PROGRAM MAIN

VAR
	bEnable: BOOL := TRUE;				(*enable or disable the functionblock by changing the value of this variable*)
	fbOcaDevice: FB_OcaDevice;			(*instance of the function block which represents the OCA Device*)
	fbOcaGain: ARRAY[E_Channel.A ..E_Channel.D] OF FB_OcaGain;	(*instances of the function block which represents the OCA Object*)

	{attribute hide}	bInit: BOOL;	(*will be TRUE after the first cycle*) 

	stRole: ARRAY[E_Channel.A ..E_Channel.D] OF ST_StringProperty;			(*structures which will contain the result 'Role' *)
	stLabel: ARRAY[E_Channel.A ..E_Channel.D] OF ST_StringProperty;			(*structures which will contain the text of the property 'Label' *)
	stGain:  ARRAY[E_Channel.A ..E_Channel.D] OF ST_Float32Property;		(*structures which will contain the value of the property 'Gain'*)
	aNewValueGain: ARRAY[E_Channel.A ..E_Channel.D] OF REAL;				(*the values which sould be set*)
	_aNewValueGain: ARRAY[E_Channel.A ..E_Channel.D] OF REAL;

	eCurrentChannel: E_Channel;		(*variable used to loop throug all channels*) 	
END_VAR

A_Init();		(*enter IP Address and other parameters of the device in this Action*)  
A_Operation();	(*calls FB_OcaDevice and the Subscription Method*) 
A_Operation1();	(*tries to get basic, inherited properties and call the method GetGain*)
A_Operation2();	(*tries to read Notifications*)
A_Operation3();	(*tries to set new 'Gain'-values*)

ACTION A_Init:
IF NOT bInit THEN
	bInit := TRUE;

	(* ----------- Init devices -------------*)
	InitDeviceList();
	fbOcaDevice.sDeviceName := 'Amplifier_2';

	fbOcaDevice.bLocalOcaDevice := FALSE;

	
	(* ----------- Init the object (assigned to a device) -------------*)
	InitOcaObjectList();
	fbOcaGain[E_Channel.A].__setsOcaObjectDescription(sOcaObjectDescription := 'Gain_A', pLink := fbOcaDevice.pLink); 
	fbOcaGain[E_Channel.B].__setsOcaObjectDescription(sOcaObjectDescription := 'Gain_B', pLink := fbOcaDevice.pLink); 
	fbOcaGain[E_Channel.C].__setsOcaObjectDescription(sOcaObjectDescription := 'Gain_C', pLink := fbOcaDevice.pLink); 
	fbOcaGain[E_Channel.D].__setsOcaObjectDescription(sOcaObjectDescription := 'Gain_D', pLink := fbOcaDevice.pLink); 
END_IF
END_ACTION

ACTION A_Operation:
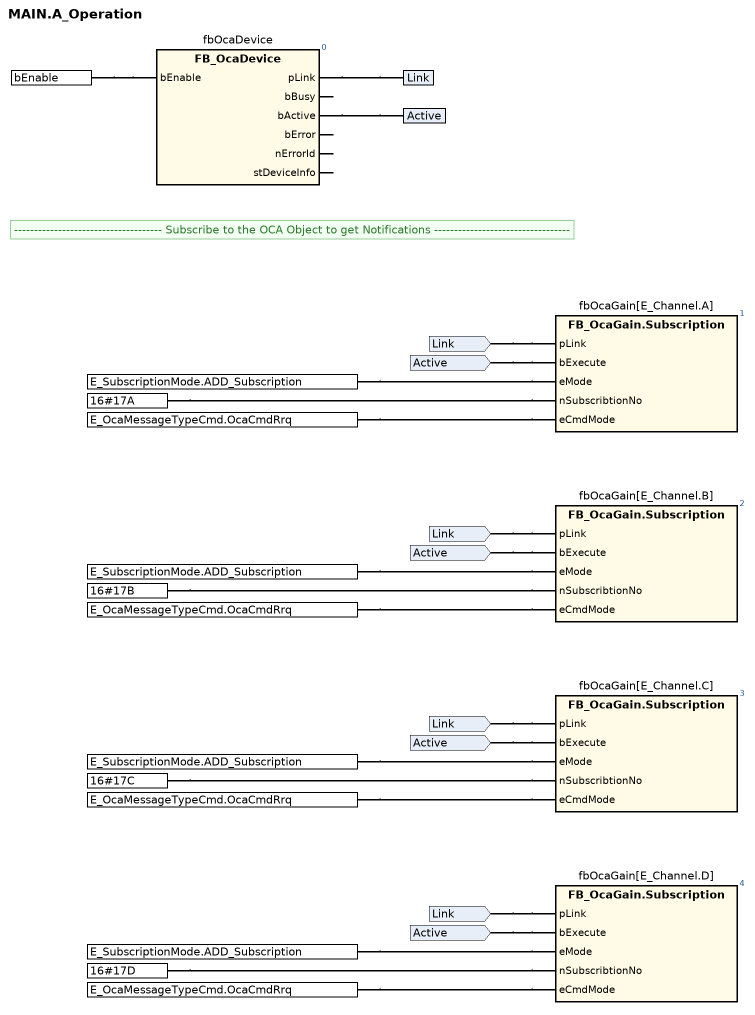
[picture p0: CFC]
fbOcaDevice(bEnable := bEnable); // FB_OcaDevice
// ------------------------------------- Subscribe to the OCA Object to get Notifications ----------------------------------
fbOcaGain[E_Channel.A].Subscription(pLink := fbOcaDevice.pLink, bExecute := fbOcaDevice.bActive, eMode := E_SubscriptionMode.ADD_Subscription, nSubscribtionNo := 16#17A, eCmdMode := E_OcaMessageTypeCmd.OcaCmdRrq);
fbOcaGain[E_Channel.B].Subscription(pLink := fbOcaDevice.pLink, bExecute := fbOcaDevice.bActive, eMode := E_SubscriptionMode.ADD_Subscription, nSubscribtionNo := 16#17B, eCmdMode := E_OcaMessageTypeCmd.OcaCmdRrq);
fbOcaGain[E_Channel.C].Subscription(pLink := fbOcaDevice.pLink, bExecute := fbOcaDevice.bActive, eMode := E_SubscriptionMode.ADD_Subscription, nSubscribtionNo := 16#17C, eCmdMode := E_OcaMessageTypeCmd.OcaCmdRrq);
fbOcaGain[E_Channel.D].Subscription(pLink := fbOcaDevice.pLink, bExecute := fbOcaDevice.bActive, eMode := E_SubscriptionMode.ADD_Subscription, nSubscribtionNo := 16#17D, eCmdMode := E_OcaMessageTypeCmd.OcaCmdRrq);
END_ACTION

ACTION A_Operation1:
(*loop to all Channels (A,B,C,D) to get the Property 'Role', the Property 'Label'  and the current value of 'Gain' - this is done just once cause of the rising edge at bExecute*)
FOR eCurrentChannel := E_Channel.A TO E_Channel.D DO
	fbOcaGain[eCurrentChannel].GetRole(
		pLink:= fbOcaDevice.pLink,						//link the OCA Object to the OCA Device
		bExecute:= fbOcaDevice.bActive);				//execute this methode when the instance of FB_OcaDevice is ready and do this just once to get the current Role of the OCA Object
	stRole[eCurrentChannel] := fbOcaGain[eCurrentChannel].stRole;	

	fbOcaGain[eCurrentChannel].GetLabel(
		pLink:= fbOcaDevice.pLink,						//link the OCA Object to the OCA Device
		bExecute:= fbOcaDevice.bActive);				//execute this methode when the instance of FB_OcaDevice is ready and do this just once to get the current Label of the OCA Object
	stLabel[eCurrentChannel] := fbOcaGain[eCurrentChannel].stLabel;	

	fbOcaGain[eCurrentChannel].GetGain(
		pLink:= fbOcaDevice.pLink,						//link the OCA Object to the OCA Device
		bExecute:= fbOcaDevice.bActive);				//execute this methode when the instance of FB_OcaDevice is ready and do this just once to get the current Label of the OCA Object
	stGain[eCurrentChannel] := fbOcaGain[eCurrentChannel].stGain;	
END_FOR
END_ACTION

ACTION A_Operation2:
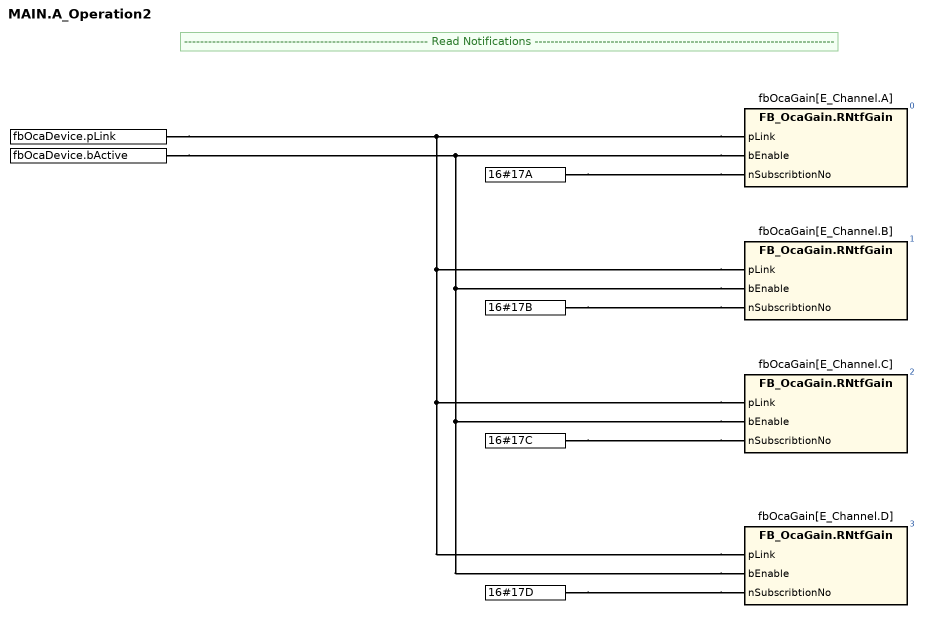
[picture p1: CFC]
// ------------------------------------------------------------- Read Notifications ---------------------------------------------------------------------------
fbOcaGain[E_Channel.A].RNtfGain(pLink := fbOcaDevice.pLink, bEnable := fbOcaDevice.bActive, nSubscribtionNo := 16#17A);
fbOcaGain[E_Channel.B].RNtfGain(pLink := fbOcaDevice.pLink, bEnable := fbOcaDevice.bActive, nSubscribtionNo := 16#17B);
fbOcaGain[E_Channel.C].RNtfGain(pLink := fbOcaDevice.pLink, bEnable := fbOcaDevice.bActive, nSubscribtionNo := 16#17C);
fbOcaGain[E_Channel.D].RNtfGain(pLink := fbOcaDevice.pLink, bEnable := fbOcaDevice.bActive, nSubscribtionNo := 16#17D);
END_ACTION

ACTION A_Operation3:
(*loop to all Channels (A,B,C,D) to possibly set new 'Gain' values*)
FOR eCurrentChannel := E_Channel.A TO E_Channel.D DO
	(*Set the Gain Property*)
	fbOcaGain[eCurrentChannel].SetGain(
		pLink:= fbOcaDevice.pLink,						//link the OCA Object to the OCA Device
		bExecute:= 
				(_aNewValueGain[eCurrentChannel] <> aNewValueGain[eCurrentChannel]) 
				AND fbOcaDevice.bActive,				//only execute this methode if the value changes
		fGain:= aNewValueGain[eCurrentChannel], 
		eCmdMode:= E_OcaMessageTypeCmd.OcaCmd);			//no response required - subscribed to get notifications! 					 
		
	
	_aNewValueGain[eCurrentChannel] := SEL(fbOcaDevice.bActive,
 											_aNewValueGain[eCurrentChannel],
											aNewValueGain[eCurrentChannel]);	 
	stGain[eCurrentChannel] := fbOcaGain[eCurrentChannel].stGain;	
END_FOR
END_ACTION

(* set parameters of the device *)
METHOD InitDeviceList
VAR
	i: INT  (0..(GVL_AES70.MAX_DEVICES - 1)) := 0;	//variable only used to count during initialization  
END_VAR

GVL_AES70.aOcaDevices[i].ipAddr := '169.254.40.175';		// the ip addres of the first device
GVL_AES70.aOcaDevices[i].ipPort := 30013;				// the port of the first device
GVL_AES70.aOcaDevices[i].sDeviceName := 'Amplifier_1';	// the unique name of the first device 

i:=i+1;
GVL_AES70.aOcaDevices[i].ipAddr := '169.254.1.7';	// the ip addres of the second device
GVL_AES70.aOcaDevices[i].ipPort := 30013;				// the port of the second device
GVL_AES70.aOcaDevices[i].sDeviceName := 'Amplifier_2';	// the unique name of the second device 

i:=i+1;
GVL_AES70.aOcaDevices[i].ipAddr := '169.254.163.144';	// the ip addres of the third device
GVL_AES70.aOcaDevices[i].ipPort := 42502;				// the port of the third device
GVL_AES70.aOcaDevices[i].sDeviceName := 'Amplifier_3';	// the unique name of the third device
END_METHOD

(* set parameters of the objects *)
METHOD InitOcaObjectList
VAR
	i: 	UINT  (0..(GVL_AES70.MAX_DEVICES - 1)) := 0;				//variable only used to count during initialization
	ii: UINT  (0..(GVL_AES70.MAX_OBJECTS_PER_DEVICE - 1)) := 0;		//variable only used to count during initialization  
END_VAR
(*Objects used by the first device*)
ii := 0;
GVL_AES70.aOcaDevices[i].aOcaObjectList[ii].nOcaObjectNr := 16#10000100;
GVL_AES70.aOcaDevices[i].aOcaObjectList[ii].nOwnerNr := 16#10001FE;
GVL_AES70.aOcaDevices[i].aOcaObjectList[ii].sDescription := 'PwrOn';
ii := ii+1;
GVL_AES70.aOcaDevices[i].aOcaObjectList[ii].nOcaObjectNr := 16#10000101;
GVL_AES70.aOcaDevices[i].aOcaObjectList[ii].nOwnerNr := 16#10001FE;
GVL_AES70.aOcaDevices[i].aOcaObjectList[ii].sDescription := 'LockCmd';
ii := ii+1;
GVL_AES70.aOcaDevices[i].aOcaObjectList[ii].nOcaObjectNr := 16#10000102;
GVL_AES70.aOcaDevices[i].aOcaObjectList[ii].nOwnerNr := 16#10001FE;
GVL_AES70.aOcaDevices[i].aOcaObjectList[ii].sDescription := 'Buzzer';
ii := ii+1;
GVL_AES70.aOcaDevices[i].aOcaObjectList[ii].nOcaObjectNr := 16#10000103;
GVL_AES70.aOcaDevices[i].aOcaObjectList[ii].nOwnerNr := 16#10001FE;
GVL_AES70.aOcaDevices[i].aOcaObjectList[ii].sDescription := 'LockScreen';
ii := ii+1;
GVL_AES70.aOcaDevices[i].aOcaObjectList[ii].nOcaObjectNr := 16#1000010F;
GVL_AES70.aOcaDevices[i].aOcaObjectList[ii].nOwnerNr := 16#10001FE;
GVL_AES70.aOcaDevices[i].aOcaObjectList[ii].sDescription := 'InputModes';
ii := ii+1;
GVL_AES70.aOcaDevices[i].aOcaObjectList[ii].nOcaObjectNr := 16#10000111;
GVL_AES70.aOcaDevices[i].aOcaObjectList[ii].nOwnerNr := 16#10001FE;
GVL_AES70.aOcaDevices[i].aOcaObjectList[ii].sDescription := 'OutputMode';
ii := ii+1;
GVL_AES70.aOcaDevices[i].aOcaObjectList[ii].nOcaObjectNr := 16#10008205;
GVL_AES70.aOcaDevices[i].aOcaObjectList[ii].nOwnerNr := 16#10002FE;
GVL_AES70.aOcaDevices[i].aOcaObjectList[ii].sDescription := 'Mute_A';
ii := ii+1;
GVL_AES70.aOcaDevices[i].aOcaObjectList[ii].nOcaObjectNr := 16#10010205;
GVL_AES70.aOcaDevices[i].aOcaObjectList[ii].nOwnerNr := 16#10002FE;
GVL_AES70.aOcaDevices[i].aOcaObjectList[ii].sDescription := 'Mute_B';
ii := ii+1;
GVL_AES70.aOcaDevices[i].aOcaObjectList[ii].nOcaObjectNr := 16#10018205;
GVL_AES70.aOcaDevices[i].aOcaObjectList[ii].nOwnerNr := 16#10002FE;
GVL_AES70.aOcaDevices[i].aOcaObjectList[ii].sDescription := 'Mute_C';
ii := ii+1;
GVL_AES70.aOcaDevices[i].aOcaObjectList[ii].nOcaObjectNr := 16#10020205;
GVL_AES70.aOcaDevices[i].aOcaObjectList[ii].nOwnerNr := 16#10002FE;
GVL_AES70.aOcaDevices[i].aOcaObjectList[ii].sDescription := 'Mute_D';
ii := ii+1;
GVL_AES70.aOcaDevices[i].aOcaObjectList[ii].nOcaObjectNr := 16#10008206;
GVL_AES70.aOcaDevices[i].aOcaObjectList[ii].nOwnerNr := 16#10002FE;
GVL_AES70.aOcaDevices[i].aOcaObjectList[ii].sDescription := 'Gain_A';
ii := ii+1;
GVL_AES70.aOcaDevices[i].aOcaObjectList[ii].nOcaObjectNr := 16#10010206;
GVL_AES70.aOcaDevices[i].aOcaObjectList[ii].nOwnerNr := 16#10002FE;
GVL_AES70.aOcaDevices[i].aOcaObjectList[ii].sDescription := 'Gain_B';
ii := ii+1;
GVL_AES70.aOcaDevices[i].aOcaObjectList[ii].nOcaObjectNr := 16#10018206;
GVL_AES70.aOcaDevices[i].aOcaObjectList[ii].nOwnerNr := 16#10002FE;
GVL_AES70.aOcaDevices[i].aOcaObjectList[ii].sDescription := 'Gain_C';
ii := ii+1;
GVL_AES70.aOcaDevices[i].aOcaObjectList[ii].nOcaObjectNr := 16#10020206;
GVL_AES70.aOcaDevices[i].aOcaObjectList[ii].nOwnerNr := 16#10002FE;
GVL_AES70.aOcaDevices[i].aOcaObjectList[ii].sDescription := 'Gain_D';


(*Copy Oca Objects defined above to the other devices*)
i:= i+1;
GVL_AES70.aOcaDevices[i].aOcaObjectList := GVL_AES70.aOcaDevices[0].aOcaObjectList;
i:= i+1;
GVL_AES70.aOcaDevices[i].aOcaObjectList := GVL_AES70.aOcaDevices[0].aOcaObjectList;
END_METHOD

END_PROGRAM
